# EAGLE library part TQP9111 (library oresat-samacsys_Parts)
RF Amplifier 1.8-2.7GHz Gn 29.8dB P1dB 32.5dBm 2 stage Source: Datasheet
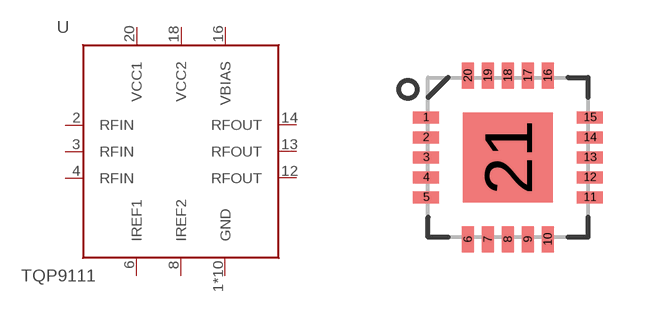
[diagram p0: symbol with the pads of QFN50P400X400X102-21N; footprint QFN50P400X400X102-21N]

Designator prefix U

## TQP9111 (DESCRIPTION: RF Amplifier 1.8-2.7GHz Gn 29.8dB P1dB 32.5dBm 2 stage; HEIGHT: 1.02mm; MFR: Qorvo; MPN: TQP9111)  [QFN50P400X400X102-21N]
1  GND  pwr
2  RFIN  in
3  RFIN  in
4  RFIN  in
5  GND  pwr
6  IREF1  pas
7  GND  pwr
8  IREF2  pas
9  GND  pwr
10  GND  pwr
11  GND  pwr
12  RFOUT  out
13  RFOUT  out
14  RFOUT  out
15  GND  pwr
16  VBIAS  pwr
17  GND  pwr
18  VCC2  pwr
19  GND  pwr
20  VCC1  pwr
21  GND  pwr

## Footprint QFN50P400X400X102-21N (pad centres in mm)
QFN-20
smd 0.65 x 0.3: 1 -2.05,1; 2 -2.05,0.5; 3 -2.05,0; 4 -2.05,-0.5; 5 -2.05,-1; 11 2.05,-1; 12 2.05,-0.5; 13 2.05,0; 14 2.05,0.5; 15 2.05,1
smd 0.3 x 0.65: 6 -1,-2.05; 7 -0.5,-2.05; 8 0,-2.05; 9 0.5,-2.05; 10 1,-2.05; 16 1,2.05; 17 0.5,2.05; 18 0,2.05; 19 -0.5,2.05; 20 -1,2.05
smd 2.25 x 2.25: 21 0,0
